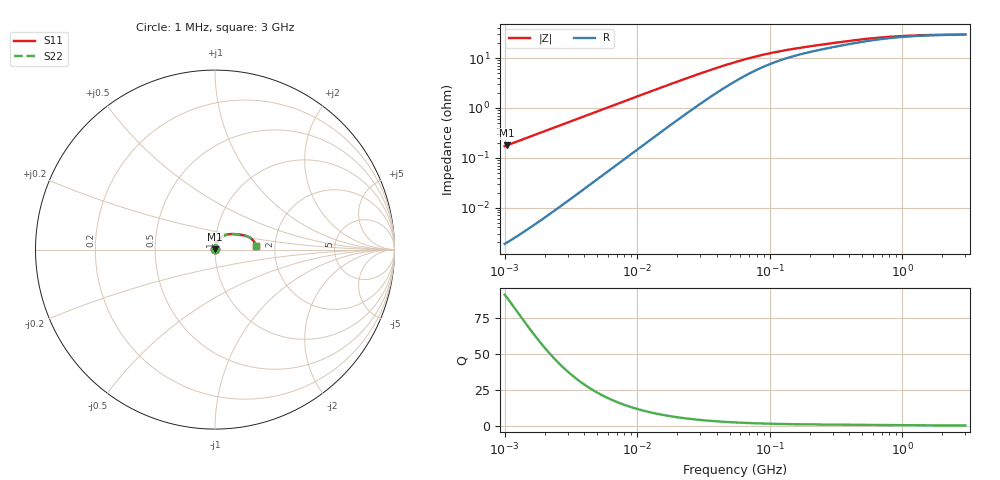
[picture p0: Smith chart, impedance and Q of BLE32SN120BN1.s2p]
! BLE32SN120BN1
# Hz S RI R 50
!Freq.(Hz) S11(Real) S11(Imag) S21(Real) S21(Imag) S12(Real) S12(Imag) S22(Real) S22(Imag)
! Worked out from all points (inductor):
!   401 points, 1 MHz to 3 GHz, reference 50 ohm
!   read as one part in series: L = 27.2 nH near 1.041 MHz
!   highest Q = 89.5 at 1.041 MHz (marker M1), where L = 27.2 nH
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1000000  2.16e-05 0.00171  1 -0.00171  1 -0.00171  2.16e-05 0.00171
1040844  2.31e-05 0.00178  1 -0.00178  1 -0.00178  2.31e-05 0.00178
3823119  0.000261 0.00653  0.9997 -0.00653  0.9997 -0.00653  0.000261 0.00653
8017732  0.00113 0.0136  0.9989 -0.0136  0.9989 -0.0136  0.00113 0.0136
1.461624e7  0.00367 0.0244  0.9963 -0.0244  0.9963 -0.0244  0.00367 0.0244
2.225279e7  0.0082 0.036  0.9918 -0.036  0.9918 -0.036  0.0082 0.036
3.127247e7  0.0153 0.0482  0.9847 -0.0482  0.9847 -0.0482  0.0153 0.0482
4.22235e7  0.0255 0.0602  0.9745 -0.0602  0.9745 -0.0602  0.0255 0.0602
5.477226e7  0.0382 0.0704  0.9618 -0.0704  0.9618 -0.0704  0.0382 0.0704
6.428402e7  0.0477 0.0759  0.9523 -0.0759  0.9523 -0.0759  0.0477 0.0759
7.544761e7  0.0582 0.0805  0.9418 -0.0805  0.9418 -0.0805  0.0582 0.0805
8.679508e7  0.068 0.0835  0.932 -0.0835  0.932 -0.0835  0.068 0.0835
1.018679e8  0.0796 0.0857  0.9204 -0.0857  0.9204 -0.0857  0.0796 0.0857
1.403209e8  0.1021 0.0868  0.8979 -0.0868  0.8979 -0.0868  0.1021 0.0868
2.094008e8  0.1281 0.085  0.8719 -0.085  0.8719 -0.085  0.1281 0.085
3.188066e8  0.1542 0.0813  0.8458 -0.0813  0.8458 -0.0813  0.1542 0.0813
4.480278e8  0.1753 0.0757  0.8247 -0.0757  0.8247 -0.0757  0.1753 0.0757
6.049187e8  0.1925 0.0676  0.8075 -0.0676  0.8075 -0.0676  0.1925 0.0676
8.005644e8  0.2056 0.058  0.7944 -0.058  0.7944 -0.058  0.2056 0.058
1.038491e9  0.2146 0.0484  0.7854 -0.0484  0.7854 -0.0484  0.2146 0.0484
1.402151e9  0.2217 0.0381  0.7783 -0.0381  0.7783 -0.0381  0.2217 0.0381
3e9  0.2295 0.0191  0.7705 -0.0191  0.7705 -0.0191  0.2295 0.0191
